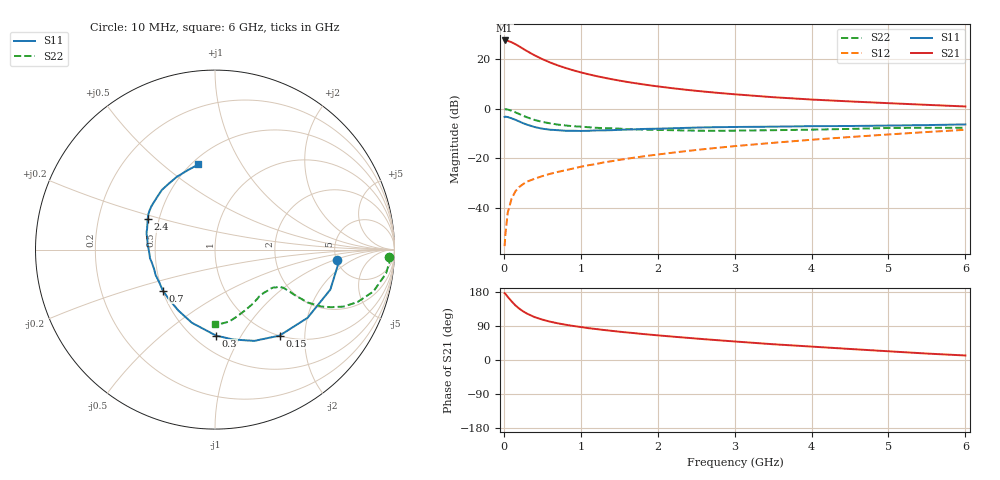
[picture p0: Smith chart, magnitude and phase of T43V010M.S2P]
! Infineon Technologies  Discrete & RF Semiconductors
! BFR182T
! Si NPN RF Bipolar Junction Transistor in SC75
! VCE = 3 V  IC = 10 mA
! Common Emitter S-Parameters:  October  1999
# GHz  S  MA  R  50
!  f  S11  S21  S12  S22
! GHz  MAG  ANG  MAG  ANG  MAG  ANG  MAG  ANG
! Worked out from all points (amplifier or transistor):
!   36 points, 10 MHz to 6 GHz, reference 50 ohm
!   highest |S21| = 27.5 dB at 10 MHz (marker M1)
!   |S21| within 3 dB of that: start of sweep to 231.9 MHz
!   unconditionally stable (mu >= 1): 987 MHz to 3.79 GHz
!   at 250 MHz: K = 0.45, MSG = 27.3 dB, |S12| = -30.4 dB
!   at 1.4 GHz: K = 1.07, MAG = 14.9 dB, |S12| = -21.1 dB
!   at 6 GHz: K = 0.84, MSG = 4.7 dB, |S12| = -8.5 dB
!   lowest NFmin = 1.50 dB at 450 MHz
!   S11 on the Smith chart (normalised r, x): 10 MHz: 5.06, -1.13; 150 MHz: 1.00, -1.50; 300 MHz: 0.63, -0.79; 700 MHz: 0.50, -0.27; 2.4 GHz: 0.43, +0.18; 6 GHz: 0.54, +0.67
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0.01  0.6838 -5.0  23.75 176.3  0.0017 80.9  0.9727 -2.3
0.02  0.6917 -6.4  23.69 174.8  0.0029 90.7  0.9782 -3.2
0.05  0.6802 -19.1  23.35 166.8  0.008 85.4  0.9622 -7.9
0.1  0.6406 -36.4  21.87 155.0  0.0153 75.4  0.9129 -14.8
0.15  0.5992 -53.1  19.99 144.2  0.0216 69.2  0.8462 -20.2
0.2  0.5537 -66.7  18.04 135.6  0.0265 66.2  0.7836 -23.9
0.25  0.511 -78.6  16.15 128.5  0.0302 61.1  0.7219 -26.4
0.3  0.4787 -89.4  14.52 122.5  0.0339 60.4  0.6733 -28.1
0.4  0.4277 -107.5  11.91 113.2  0.0388 57.6  0.5944 -29.7
0.5  0.3962 -121.0  10.01 106.6  0.0439 58.1  0.5434 -29.7
0.6  0.3776 -132.6  8.561 101.2  0.0487 59.3  0.5074 -29.7
0.7  0.3695 -141.8  7.485 96.9  0.0532 60.0  0.4796 -29.4
0.9  0.3599 -156.8  5.953 89.9  0.0623 61.9  0.4439 -29.2
1.1  0.3594 -168.5  4.948 84.0  0.0727 63.7  0.4237 -29.7
1.3  0.3668 -177.1  4.233 79.2  0.083 64.7  0.4066 -30.7
1.6  0.3798 172.6  3.472 72.7  0.0983 65.8  0.3895 -32.7
2.2  0.4039 158.8  2.581 61.6  0.1304 66.6  0.3691 -39.1
2.4  0.4125 155.4  2.381 58.3  0.1416 66.5  0.363 -41.7
3.5  0.4349 138.3  1.707 41.6  0.2055 63.8  0.3693 -56.7
4.5  0.4486 125.2  1.403 29.1  0.269 59.3  0.3922 -71.7
5.5  0.4679 108.9  1.197 17.0  0.3394 53.8  0.4135 -84.6
6  0.4833 101.0  1.11 11.9  0.3763 50.2  0.4133 -89.9
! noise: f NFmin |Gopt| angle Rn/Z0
0.45  1.5  0.26  43  0.28
0.9  1.6  0.24  87  0.22
1.8  2.1  0.2  170  0.2
